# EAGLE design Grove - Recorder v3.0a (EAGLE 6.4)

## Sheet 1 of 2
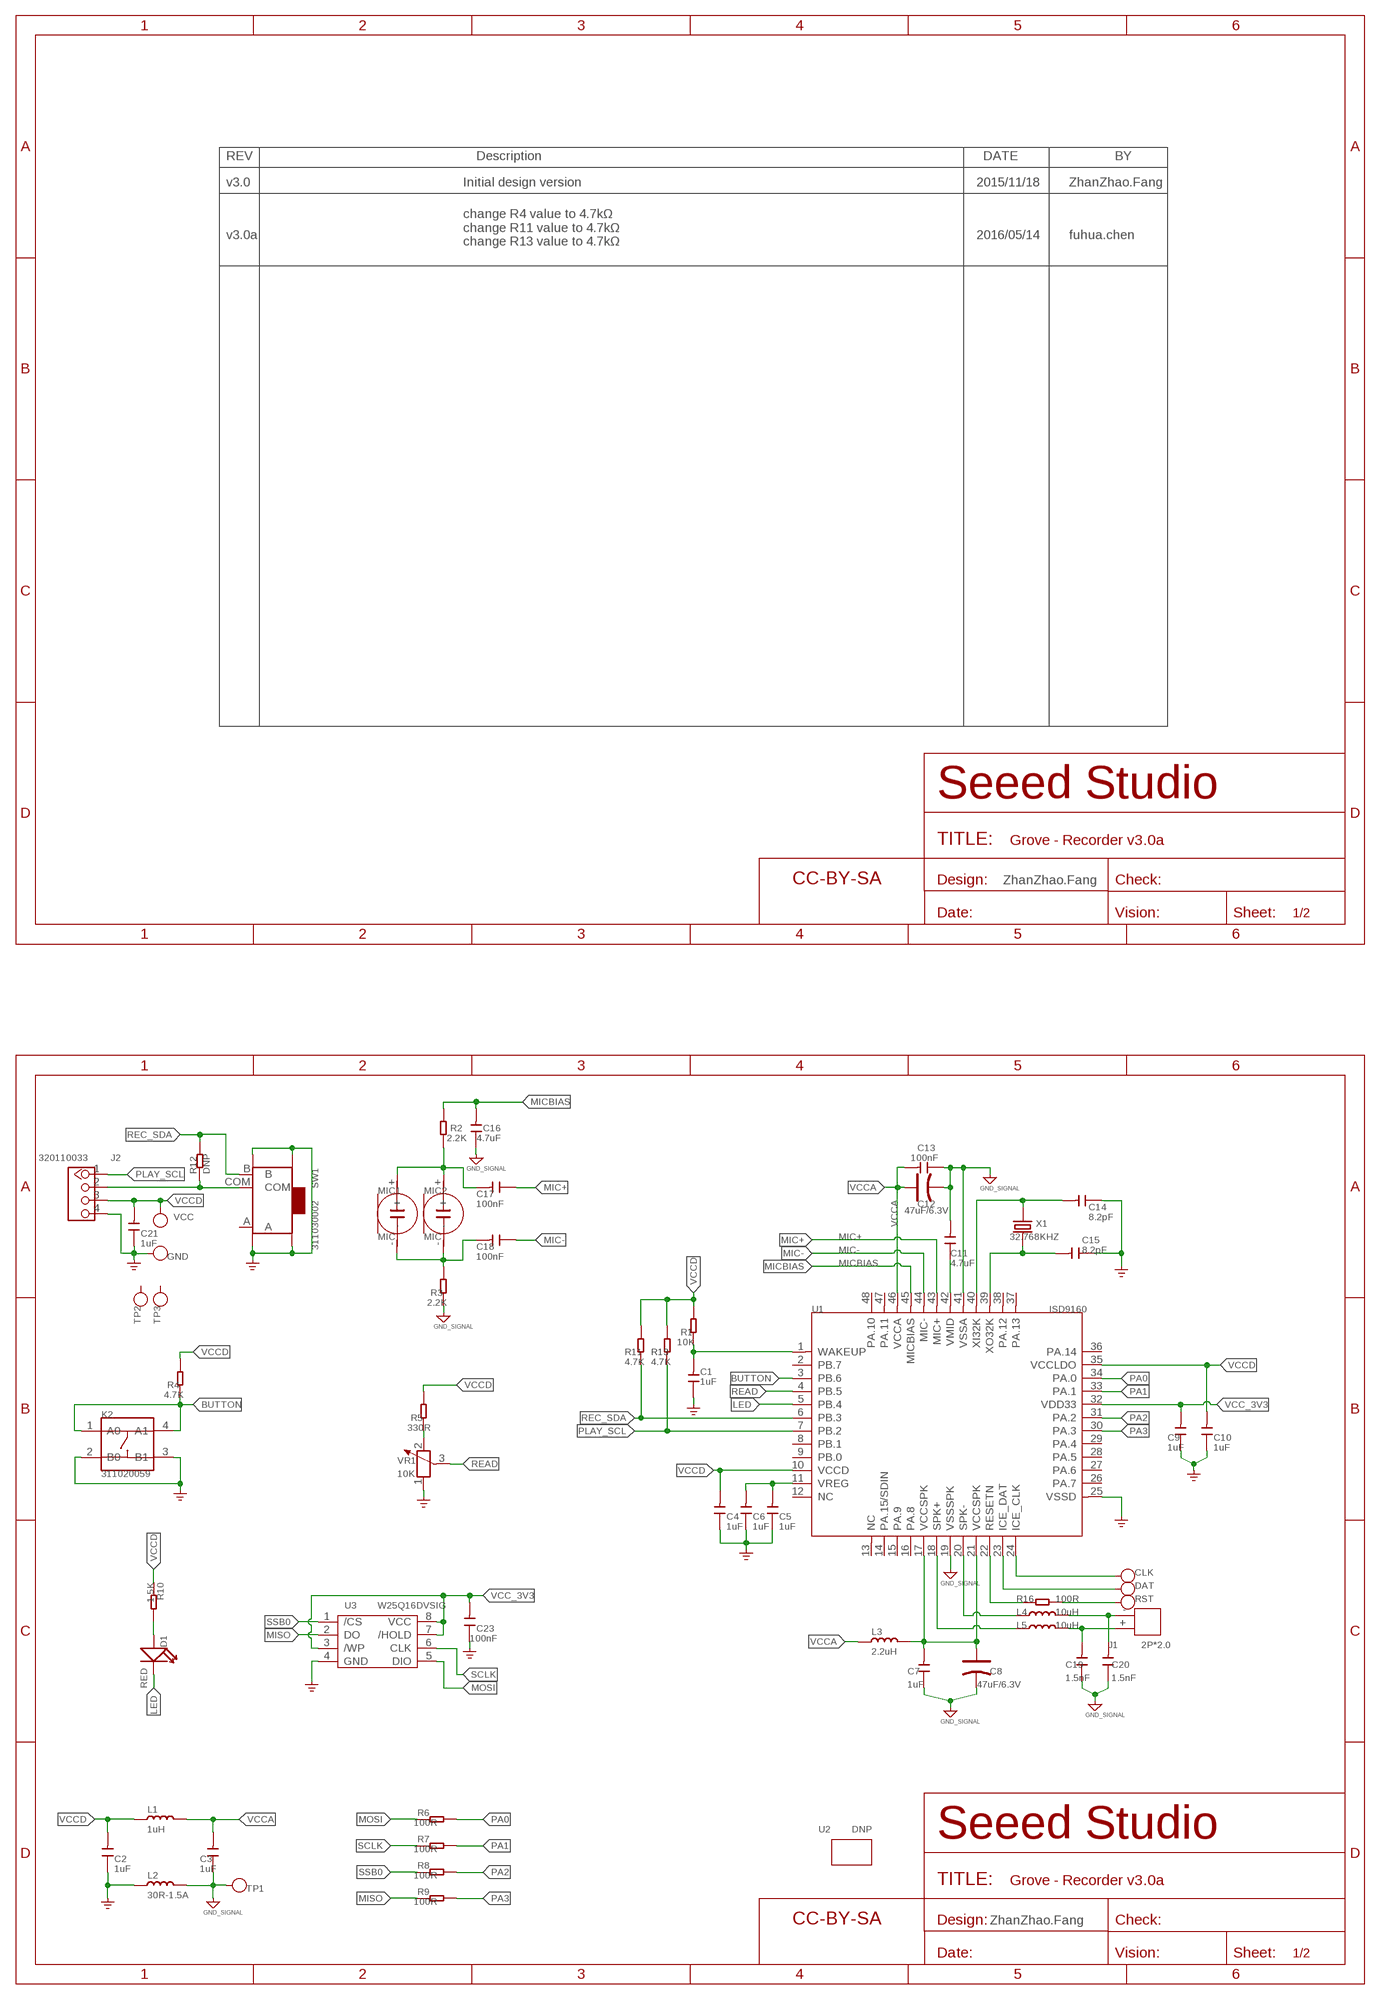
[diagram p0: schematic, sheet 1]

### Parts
C1  1uF  CAP-0603  [C0603]
C2  1uF  CAP-0603  [C0603]
C3  1uF  CAP-0603  [C0603]
C4  1uF  CAP-0603  [C0603]
C5  1uF  CAP-0603  [C0603]
C6  1uF  CAP-0603  [C0603]
C7  1uF  CAP-0603  [C0603]
C8  47uF/6.3V  CAP-POLAR-AVX-A  [AVX-A]
C9  1uF  CAP-0603  [C0603]
C10  1uF  CAP-0603  [C0603]
C11  4.7uF  CAP-0805  [C0805]
C12  47uF/6.3V  CAP-POLAR-AVX-A  [AVX-A]
C13  100nF  CAP-0402  [C0402]
C14  8.2pF  CAP-0402  [C0402]
C15  8.2pF  CAP-0402  [C0402]
C16  4.7uF  CAP-0805  [C0805]
C17  100nF  CAP-0402  [C0402]
C18  100nF  CAP-0402  [C0402]
C19  1.5nF  CAP-0402  [C0402]
C20  1.5nF  CAP-0402  [C0402]
C21  1uF  CAP-0603  [C0603]
C23  100nF  CAP-0402  [C0402]
CLK  DNP  TEST-POINT'4545'  [TP-D45MIL]
D1  RED  LED'RIGHT'  [LED-SIDE-VIEW-0603-RIGHT]
DAT  DNP  TEST-POINT'4545'  [TP-D45MIL]
FR1  DNP  SEEEDSTUDIO-OPEN-SCH-FRAME  [SEEEDSTUDIO-PCB-FRAME]
FR2  DNP  SEEEDSTUDIO-OPEN-SCH-FRAME  [SEEEDSTUDIO-PCB-FRAME]
GND  DNP  TEST-POINT'4545'  [TP-D45MIL]
J1  2P*2.0  JST-2P-DIP'2.0'  [H2-2.0-6X4.5MM]
J2  320110033  GROVE-CONNECTOR-DIP-2.0  [HW4-2.0]
K2  311020059  BUTTON-4P'TS-1109'  [SW4-6.0X6.0X5.0MM]
L1  1uH  INDUCTOR/FERRITE-BEAD'0805'  [L0805]
L2  30R-1.5A  INDUCTOR/FERRITE-BEAD'0603'  [L0603]
L3  2.2uH  INDUCTOR/FERRITE-BEAD'0805'  [L0805]
L4  10uH  INDUCTOR/FERRITE-BEAD'0805'  [L0805]
L5  10uH  INDUCTOR/FERRITE-BEAD'0805'  [L0805]
MIC1  MIC  MIC-2P'EAO-9745-PFA-C1033-28-008'  [MIC2-D9.7XH4.5MM]
MIC2  MIC  MIC-2P'EAO-9745-PFA-C1033-28-008'  [MIC2-D9.7XH4.5MM]
R1  10K  RES-0402  [R0402]
R2  2.2K  RES-0402  [R0402]
R3  2.2K  RES-0402  [R0402]
R4  4.7K  RES-0402  [R0402]
R5  330R  RES-0402  [R0402]
R6  100R  RES-0402  [R0402]
R7  100R  RES-0402  [R0402]
R8  100R  RES-0402  [R0402]
R9  100R  RES-0402  [R0402]
R10  1.5K  RES-0402  [R0402]
R11  4.7K  RES-0402  [R0402]
R12  DNP  RES-0402  [R0402]
R13  4.7K  RES-0402  [R0402]
R16  100R  RES-0402  [R0402]
RST  DNP  TEST-POINT'4545'  [TP-D45MIL]
SW1  311030002  SWITCH-3+4P  [SW7-SMD-L6.7X2.7X3.2MM]
TP1  DNP  TEST-POINT'4545'  [TP-D45MIL]
TP2  DNP  TEST-POINT'4545'  [TP-D45MIL]
TP3  DNP  TEST-POINT'4545'  [TP-D45MIL]
U1  ISD9160  MCU-ISD9160  [LQFP48-0.5-7X7MM]
U2  DNP  GROVE'2U'  [GROVE-1*2-TEST-PLATFORM]
U3  W25Q16DVSIG  FLASH-W25X80  [SOIC8-1.27-5.3X5.3MM]
VCC  DNP  TEST-POINT'4545'  [TP-D45MIL]
VR1  10K  RES-ADJ-SX3362P  [ADJR3-7.0X7.0X5.0MM]
X1  32.768KHZ  CRYSTAL-2P-3215  [X2-SMD-3.2X1.5X0.55MM]

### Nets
AGND: C3.1 C7.1 C8.- C11.2 C12.- C13.1 C16.1 C19.1 C20.1 L2.2 R3.1 TP1.T U1.19(VSSSPK) U1.41(VSSA) ; supply symbol labelled GND_SIGNAL
BUTTON: K2.1(A0) K2.4(A1) R4.1 U1.3(PB.6)
GND: C1.1 C2.1 C4.1 C5.1 C6.1 C9.1 C10.1 C14.1 C15.1 C21.1 C23.1 GND.T J2.4 K2.2(B0) K2.3(B1) L2.1 SW1.SS1 SW1.SS2 SW1.SS3 SW1.SS4 U1.25(VSSD) U3.4(GND) VR1.1 ; supply symbol labelled GND_POWER
ICE_CLK: CLK.T U1.24(ICE_CLK)
LED: D1.2(-) U1.5(PB.4)
MIC+: C17.1 U1.43(MIC+)
MIC-: C18.1 U1.44(MIC-)
MICBIAS: C16.2 R2.2 U1.45(MICBIAS)
MISO: R9.2 U3.2(DO)
MOSI: R6.2 U3.5(DIO)
N$1: C1.2 R1.1 U1.1(WAKEUP)
N$2: C7.2 C8.+ L3.2 U1.17(VCCSPK) U1.21(VCCSPK)
N$3: C5.2 C6.2 U1.11(VREG)
N$4: C11.1 U1.42(VMID)
N$5: C17.2 MIC1.+ MIC2.+ R2.1
N$6: D1.1(+) R10.1
N$7: C14.2 U1.40(XI32K) X1.1
N$8: C15.2 U1.39(XO32K) X1.2
N$9: C18.2 MIC1.- MIC2.- R3.2
N$10: J2.2 R12.2 SW1.COM
N$11: R5.1 VR1.2
N$12: DAT.T U1.23(ICE_DAT)
N$13: L4.1 U1.20(SPK-)
N$16: R16.2 U1.22(RESETN)
N$17: R16.1 RST.T
N$23: L5.1 U1.18(SPK+)
N$24: C20.2 J1.- L4.2
N$25: C19.2 J1.+ L5.2
PA0: R6.1 U1.34(PA.0)
PA1: R7.1 U1.33(PA.1)
PA2: R8.1 U1.31(PA.2)
PA3: R9.1 U1.30(PA.3)
PLAY_SCL: J2.1 R13.1 U1.7(PB.2)
READ: U1.4(PB.5) VR1.3
REC_SDA: R11.1 R12.1 SW1.B U1.6(PB.3)
SCLK: R7.2 U3.6(CLK)
SSB0: R8.2 U3.1(/CS)
VCC_3V3: C9.2 C23.2 U1.32(VDD33) U3.3(/WP) U3.7(/HOLD) U3.8(VCC)
VCCA: C3.2 C12.+ C13.2 L1.2 L3.1 U1.46(VCCA)
VCCD: C2.2 C4.2 C10.2 C21.2 J2.3 L1.1 R1.2 R4.2 R5.2 R10.2 R11.2 R13.2 U1.10(VCCD) U1.35(VCCLDO) VCC.T
Unconnected: SW1.A TP2.T TP3.T U1.2(PB.7) U1.8(PB.1) U1.9(PB.0) U1.12(NC) U1.13(NC) U1.14(PA.15/SDIN) U1.15(PA.9) U1.16(PA.8) U1.26(PA.7) U1.27(PA.6) U1.28(PA.5) U1.29(PA.4) U1.36(PA.14) U1.37(PA.13) U1.38(PA.12) U1.47(PA.11) U1.48(PA.10)

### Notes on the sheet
- v3.0 | Initial design version | 2015/11/18 | ZhanZhao.Fang
- v3.0a | 2016/05/14 | fuhua.chen
- change R4 value to 4.7kΩ
  change R11 value to 4.7kΩ
  change R13 value to 4.7kΩ
- ZhanZhao.Fang
- ZhanZhao.Fang

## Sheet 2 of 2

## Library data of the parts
C1-C7 C9-C11 C13-C21 C23 = Discrete-new:CAP: Ceramic Capacitors
C8 C12 = Discrete-new:CAP-POLAR: Electrolytic Capacitors,Tantalum Capacitors and Super Capacitors
CLK DAT GND RST TP1-TP3 VCC = Discrete-new:TEST-POINT; PARTNO: DNP
D1 = Discrete-new:LED
FR1 FR2 = moudle-new:SEEEDSTUDIO-OPEN-SCH-FRAME
J1 = Connector-new:JST-2P-DIP: 2P-2.0:320110049;2P-2.0-90D:320110027;2P-2.54:320110053;2P-2.54-90D:320110000
J2 = Connector-new:GROVE-CONNECTOR-DIP: 4P-2.0:320110033;4P-2.0-90D:320110034
K2 = Discrete-new:BUTTON-4P: SW4-6.0X6.0X5.0MM:311020024;SW4-8.0X8.0X9.0MM:311020028;SW4-SMD-6.0X6.0X5.0MM:311020004;SW4-SMD-3.35X3.35X1.5MM:311020030;SW4-SMD-5.2X5.2X2.5MM:311020046
L1-L5 = Discrete-new:INDUCTOR/FERRITE-BEAD
MIC1 MIC2 = Discrete-new:MIC-2P: 312030029
R1-R13 R16 = Discrete-new:RES
SW1 = Discrete-new:SWITCH-3+4P: SW7-SMD-6.7X2.6X1.4MM-90D:311030002;SW7-SMD-L6.7X2.7X3.2MM:311030001
U1 = template:MCU-ISD9160
U2 = moudle-new:GROVE
U3 = IC-new:FLASH-W25X80: 1M-BIT,2M-BIT,4M-BIT AND 8M-BIT SERIAL FLASH MEMORY WITH 4KB SECTORS AND DUAL OUTPUT SPI
VR1 = Discrete-new:RES-ADJ: Potentiometer
X1 = Discrete-new:CRYSTAL-2P

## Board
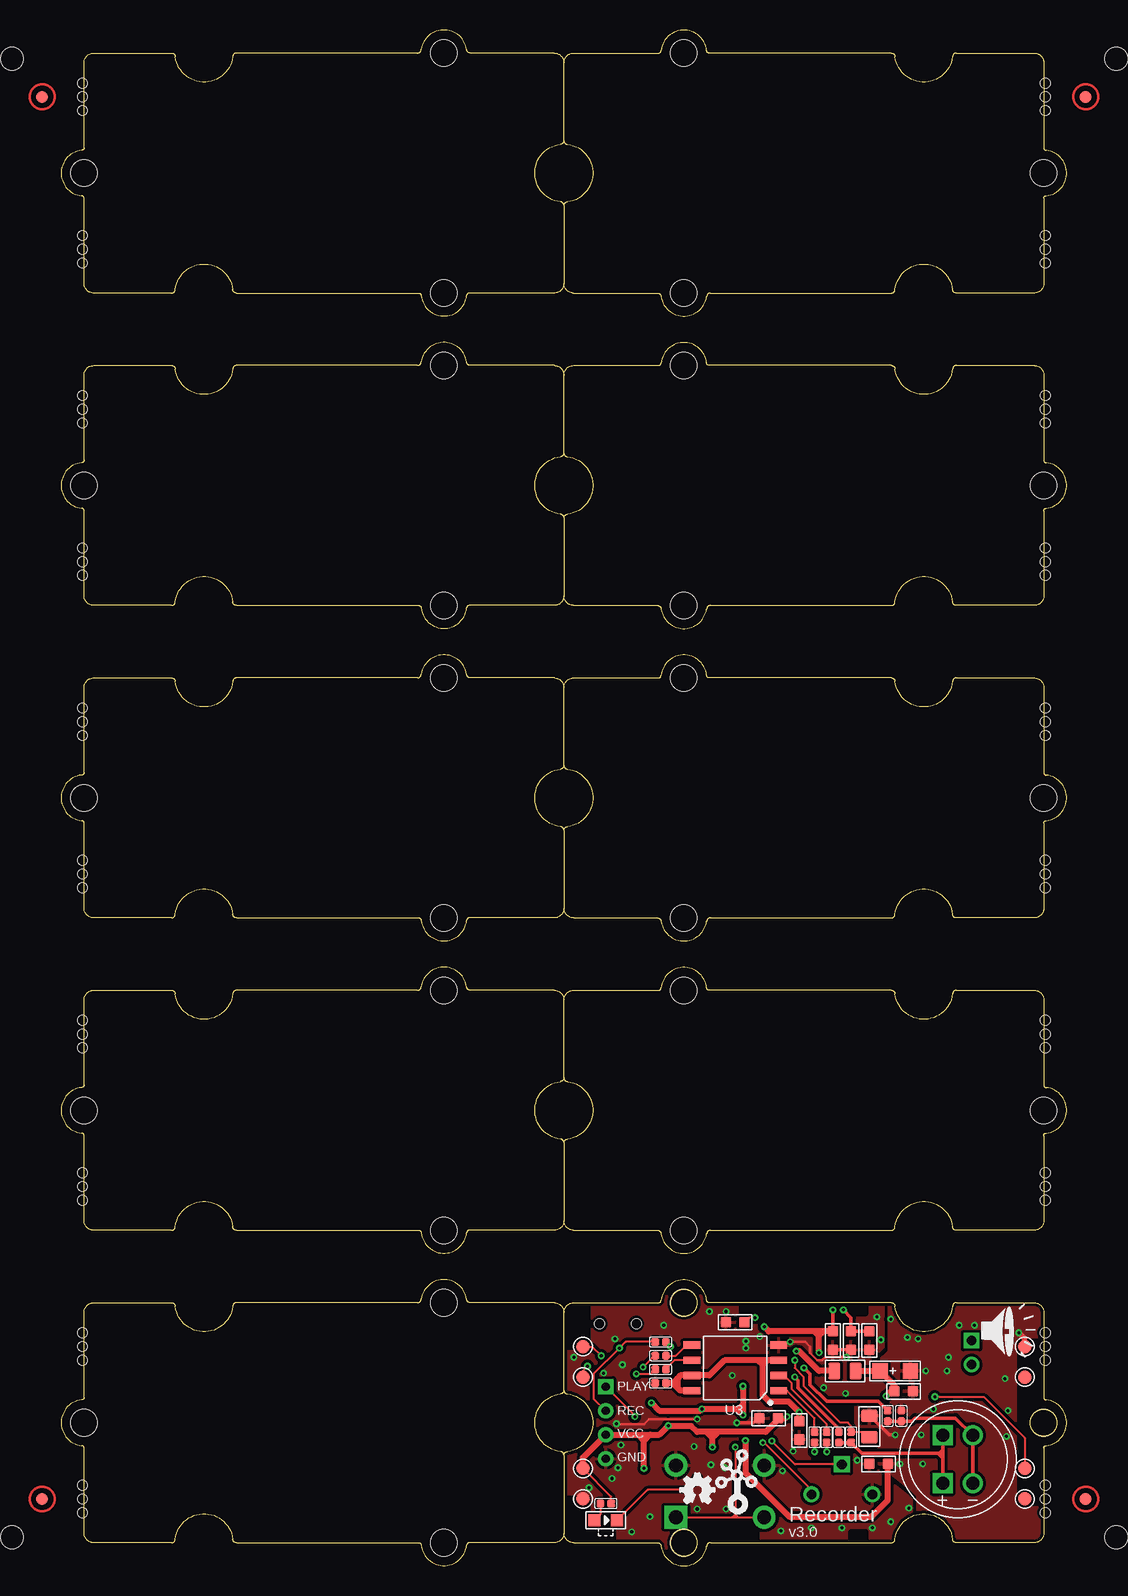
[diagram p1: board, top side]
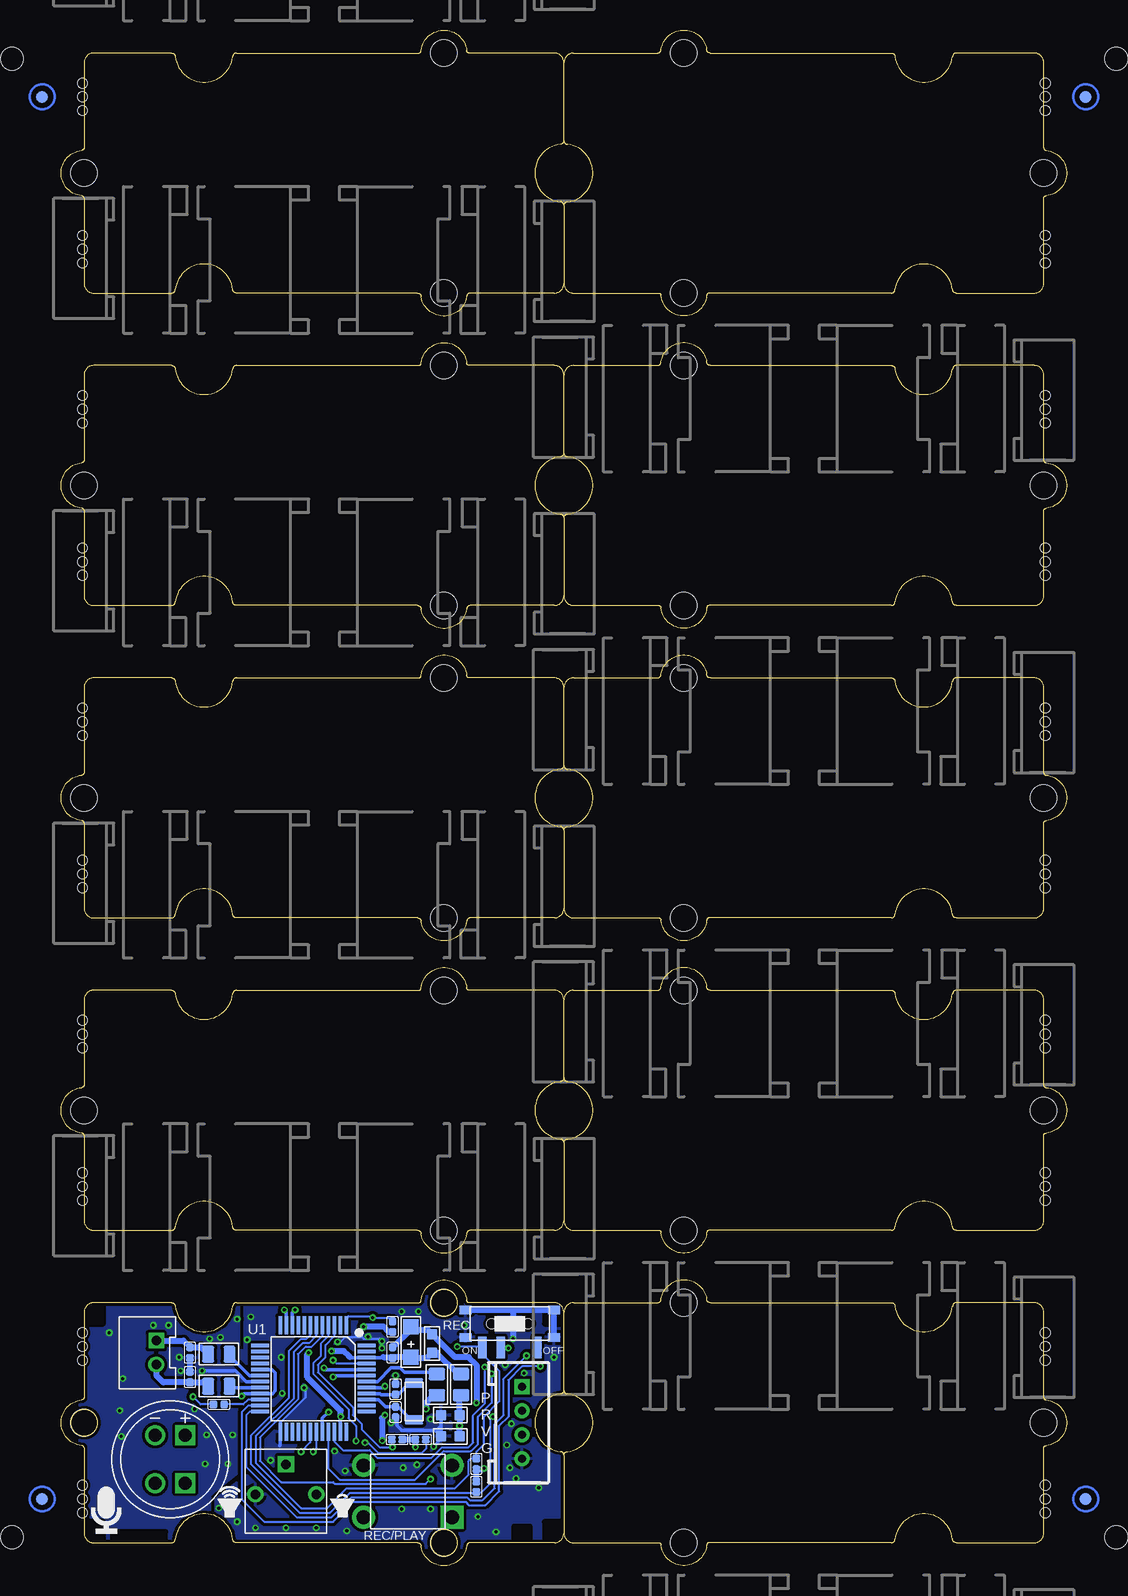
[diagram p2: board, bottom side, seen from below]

Size 83.82 x 127.98 mm. Coordinates in mm from the lower left corner, seen from the top.
Copper layers (1*16): Top 0.035mm / dielectric 1.5mm / Bottom 0.035mm
Design rules "SeeedStudio_2layer_DRU_no_angle_20140221 *": minimum track width 6mil, minimum drill 10mil, track to track 6mil, track to pad 6mil, pad to pad 6mil, via to via 6mil, smd to smd 0mil, copper to edge 10mil, drill to drill 10mil, minimum pad ring 10mil, minimum via ring 6mil, stop-mask expansion 2mil, vias tented up to drill 25mil, thermal gap 10mil
Holes 0.8 mm at 1.78,4.43 1.78,6.71 1.78,5.57 1.78,17.13 1.78,19.41 1.78,18.27 1.78,30.46 1.78,32.75 1.78,31.61 1.78,43.16 1.78,45.45 1.78,44.31 1.78,56.5 1.78,58.78 1.78,57.64 1.78,69.2 1.78,71.48 1.78,70.34 1.78,82.53 1.78,84.82 1.78,83.68 1.78,95.23 1.78,97.52 1.78,96.38 1.78,108.57 1.78,110.85 1.78,109.71 1.78,121.27 1.78,123.55 1.78,122.41 82.04,6.71 82.04,4.43 82.04,5.57 82.04,19.41 82.04,17.13 82.04,18.27 82.04,32.75 82.04,30.46 82.04,31.61 82.04,45.45 82.04,43.16 82.04,44.31 82.04,58.78 82.04,56.5 82.04,57.64 82.04,71.48 82.04,69.2 82.04,70.34 82.04,84.82 82.04,82.53 82.04,83.68 82.04,97.52 82.04,95.23 82.04,96.38 82.04,110.85 82.04,108.57 82.04,109.71 82.04,123.55 82.04,121.27 82.04,122.41
Holes 1.91 mm at -4.13,125.59 87.95,125.59 87.95,2.4 -4.13,2.4
tRestrict: area 44.8,2 to 46,3.3
bRestrict: area 44.8,2 to 46,3.3

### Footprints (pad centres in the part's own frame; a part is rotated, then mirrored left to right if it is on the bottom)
C0603 = smd 0.889 x 0.889: 1 0,0.762; 2 0,-0.762
AVX-A = smd 1.27 x 1.27: + -1.27,0; - 1.27,0
C0805 = smd 1.397 x 1.016: 1 0,0.889; 2 0,-0.889
C0402 = smd 0.635 x 0.635: 1 0,0.445; 2 0,-0.445
TP-D45MIL = smd 1.143 x 1.143: T 0,0
LED-SIDE-VIEW-0603-RIGHT = smd 1 x 1: 1 0,-0.95; 2 0,0.95
H2-2.0-6X4.5MM = drill 0.8 pad 1.3 square: + -1,0.75 | drill 0.8 pad 1.3: - 1,0.75
HW4-2.0 = drill 0.7 pad 1.27 square: 1 -3,0 | drill 0.7 pad 1.27: 2 -1,0; 3 1,0; 4 3,0
SW4-6.0X6.0X5.0MM = drill 1.143 pad 1.905 square: 1 -3.683,2.159 | drill 1.143 pad 1.905: 2 -3.683,-2.159; 3 3.683,-2.159; 4 3.683,2.159
L0805 = smd 1.016 x 1.397: 1 -0.889,0; 2 0.889,0
L0603 = smd 0.889 x 0.889: 1 -0.762,0; 2 0.762,0
MIC2-D9.7XH4.5MM = drill 1.1 square: + 1.25,2 | drill 1.1: - -1.25,2
ROUND-MARK-1.0 = smd 1.016 x 1.016: P$1 0,0
R0402 = smd 0.635 x 0.635: 1 0,0.445; 2 0,-0.445
SW7-SMD-L6.7X2.7X3.2MM = smd 1.8 x 0.7: A 1.978,2.286; B 1.978,-2.286; COM 1.978,-0.762 | smd 0.7 x 1.016: SS1 -1.15,-3.683; SS2 1.15,-3.683; SS3 1.15,3.683; SS4 -1.15,3.683 | hole 0.813: 0,-1.524; 0,1.524
LQFP48-0.5-7X7MM = smd 1.5 x 0.3: 1 -4.45,2.75; 2 -4.45,2.25; 3 -4.45,1.75; 4 -4.45,1.25; 5 -4.45,0.75; 6 -4.45,0.25; 7 -4.45,-0.25; 8 -4.45,-0.75; 9 -4.45,-1.25; 10 -4.45,-1.75; 11 -4.45,-2.25; 12 -4.45,-2.75; 25 4.45,-2.75; 26 4.45,-2.25; 27 4.45,-1.75; 28 4.45,-1.25; 29 4.45,-0.75; 30 4.45,-0.25; 31 4.45,0.25; 32 4.45,0.75; 33 4.45,1.25; 34 4.45,1.75; 35 4.45,2.25; 36 4.45,2.75 | smd 0.3 x 1.5: 13 -2.75,-4.45; 14 -2.25,-4.45; 15 -1.75,-4.45; 16 -1.25,-4.45; 17 -0.75,-4.45; 18 -0.25,-4.45; 19 0.25,-4.45; 20 0.75,-4.45; 21 1.25,-4.45; 22 1.75,-4.45; 23 2.25,-4.45; 24 2.75,-4.45; 37 2.75,4.45; 38 2.25,4.45; 39 1.75,4.45; 40 1.25,4.45; 41 0.75,4.45; 42 0.25,4.45; 43 -0.25,4.45; 44 -0.75,4.45; 45 -1.25,4.45; 46 -1.75,4.45; 47 -2.25,4.45; 48 -2.75,4.45
GROVE-1*2-TEST-PLATFORM = hole 2.2: 10.635,10; 10.635,-10; -19.365,0
SOIC8-1.27-5.3X5.3MM = smd 0.62 x 1.4: 1 -1.905,-3.623; 2 -0.635,-3.623; 3 0.635,-3.623; 4 1.905,-3.623; 5 1.905,3.623; 6 0.635,3.623; 7 -0.635,3.623; 8 -1.905,3.623
GROVE-TEST-PLATFORM = hole 2.2: -10,-10; -10,10; 20,0
ADJR3-7.0X7.0X5.0MM = drill 0.8 pad 1.35: 1 -2.54,-0.25; 2 2.54,-0.25 | drill 0.8 pad 1.35 square: 3 0,2.25
X2-SMD-3.2X1.5X0.55MM = smd 0.762 x 1.524: 1 -1.524,0; 2 1.524,0

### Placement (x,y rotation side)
C1  56.2,20.3 90 top
C2  51.37,12.56 90 bottom
C3  52.9,18.53 0 bottom
C4  64.33,18.78 180 top
C5  67.37,18.78 180 top
C6  65.85,18.78 180 top
C7  70.23,14.52 270 top
C8  69.53,16.24 0 top
C9  61.53,11.29 180 top
C10  58.99,12.3 90 top
C11  52.52,15.1 0 bottom
C12  54.67,18.65 90 bottom
C13  56.2,17.76 0 bottom
C14  55.94,14.72 0 bottom
C15  55.94,12.81 180 bottom
C16  67.37,11.6 0 top
C17  64.83,10.71 0 top
C18  68.9,12.49 0 top
C19  73.09,17.76 180 bottom
C20  73.09,15.73 0 bottom
C21  51.37,10.78 90 bottom
C23  49.98,15.22 90 top
CLK  43.5,18.27 0 top
D1  45.4,3.79 270 top
DAT  43.5,15.73 0 top
FR1  not placed on the board
FR2  not placed on the board
GND  43.5,5.57 0 top
J1  76.65,17.76 270 bottom
J2  45.4,11.92 270 bottom
K2  54.93,6.21 180 bottom
L1  50.48,15.1 90 bottom
L2  68.14,8.49 0 top
L3  65.34,16.24 0 top
L4  70.68,14.97 180 bottom
L5  70.68,17.64 180 bottom
MIC1  74.74,8.87 0 bottom
MIC2  74.74,8.87 180 top
P1  [ROUND-MARK-1.0]  -1.59,122.41 180 bottom
P2  [ROUND-MARK-1.0]  85.41,122.41 180 bottom
P3  [ROUND-MARK-1.0]  -1.59,5.57 180 bottom
P4  [ROUND-MARK-1.0]  85.41,5.57 180 bottom
P5  [ROUND-MARK-1.0]  -1.59,122.41 180 top
P6  [ROUND-MARK-1.0]  85.41,122.41 180 top
P7  [ROUND-MARK-1.0]  85.41,5.57 180 top
P8  [ROUND-MARK-1.0]  -1.59,5.57 180 top
R1  56.2,19.92 0 bottom
R2  65.85,10.71 180 top
R3  70.04,12.49 0 top
R4  55.82,10.52 90 bottom
R5  53.86,10.52 270 bottom
R6  49.98,17.51 90 top
R7  49.98,16.37 90 top
R8  62.8,10.71 180 top
R9  63.82,10.71 180 top
R10  45.4,5.19 90 top
R11  49.21,8.49 0 bottom
R12  49.98,18.65 270 top
R13  49.21,6.59 180 bottom
R16  70.68,13.45 90 bottom
RST  80.33,8.11 0 top
SW1  46.42,20.18 270 bottom
TP1  80.33,18.27 0 top
TP2  80.33,15.73 0 top
TP3  80.33,5.57 0 top
U1  62.8,15.6 270 bottom
U2  62.55,11.92 0 bottom
U3  56.2,16.49 90 top
U4  [GROVE-TEST-PLATFORM]  61.91,90.03 180 bottom
U5  [GROVE-TEST-PLATFORM]  21.91,90.03 0 bottom
U6  [GROVE-TEST-PLATFORM]  61.91,63.99 180 bottom
U7  [GROVE-TEST-PLATFORM]  21.91,63.99 0 bottom
U8  [GROVE-TEST-PLATFORM]  61.91,37.96 180 bottom
U9  [GROVE-TEST-PLATFORM]  21.91,37.96 0 bottom
U10  [GROVE-TEST-PLATFORM]  21.91,11.92 0 bottom
U11  [GROVE-TEST-PLATFORM]  61.91,11.92 180 bottom
U12  [GROVE-TEST-PLATFORM]  61.91,116.06 180 bottom
U13  [GROVE-TEST-PLATFORM]  21.91,116.06 0 bottom
U$20  [TWIGLOGO_SMALL]  54.17,4.17 0 top
U$21  [OSHW_FILLX100_NOTEXT]  51.63,5.19 0 top
VCC  43.5,8.11 0 top
VR1  65.09,6.21 0 bottom
X1  54.42,13.7 270 bottom

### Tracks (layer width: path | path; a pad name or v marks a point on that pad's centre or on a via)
AGND  (via drill 0.25 pad 0.51)
  Top 0.305: C16.1 67.44,12.49 69.03,10.91 v69.53,10.91
  Top 0.406: TP1.T 80.33,18.91 v79.82,19.41
  Top 0.508: v56.83,14.97 56.83,13.45 | 56.83,13.45 v56.83,12.56 56.33,13.06 | 56.33,13.06 v53.4,13.06 53.28,12.94 49.85,12.94 v49.21,13.57 | 56.33,13.06 56.45,13.06 56.83,13.45 | v57.05,10.44 57.05,7.77 60.77,4.05 67.5,4.05 68.9,5.44 L2.2
  Bottom 0.305: U1.41 56.95,14.85 v56.83,14.97 | U1.19 68.39,15.35 69.28,16.24 v72.07,16.24
  Bottom 0.508: C20.1 C19.1 | C13.1 56.13,18.21 54.67,19.67 | C12.- 54.67,19.67 | v56.83,12.56 57.09,12.3 57.09,10.47 v57.05,10.44 | C11.2 52.77,14.21 53.4,13.57 v53.4,13.06 | 54.67,19.67 53.28,19.67 C3.1 50.99,17.38 49.85,17.38 49.21,16.75 v49.21,13.57
  other vias: 78.8,10.78 78.93,12.94 78.68,15.6 76.14,20.05 74.87,20.05 71.44,18.91 70.55,19.03 69.15,20.56 73.85,16.24 73.98,17.38 72.71,13.06 69.91,8.49 71.69,10.91 71.82,8.49
  pour Top (isolate 0.254, rank 2): 82.23,22.46 69.03,22.46 69.03,17.89 68.14,17 66.74,17 66.23,16.49 66.23,10.06 71.06,6.21 71.44,5.83 71.44,1 71.57,0.87 81.6,0.87 82.23,1.51
  pour Bottom (isolate 0.254, rank 2): 82.23,22.46 69.03,22.46 69.03,17.89 68.14,17 66.74,17 66.23,16.49 66.23,10.06 71.06,6.21 71.44,5.83 71.44,1 71.57,0.87 81.6,0.87 82.23,1.51
BUTTON  (via drill 0.25 pad 0.51)
  Top 0.152: v56.2,9.89 56.2,4.3 | 56.2,4.3 56.2,4.05 | K2.1 55.94,4.05 | 55.94,4.05 56.2,4.05 | 56.2,4.05 56.45,4.05 | 56.45,4.05 K2.4 | 56.45,4.05 56.2,4.3 | 56.2,4.3 55.94,4.05
  Bottom 0.152: U1.3 61.05,19.13 61.79,18.4 61.79,17.38 62.42,16.75 62.42,16.11 59.5,13.19 59.5,12.56 58.74,11.79 58.74,11.34 57.29,9.89 v56.2,9.89 56.26,9.95 R4.1
GND  (via drill 0.25 pad 0.51)
  Top 0.203: v53.02,12.23 49.01,12.23 48.58,11.79 46.34,11.79 v46.29,11.85 | v60.77,18.65 62.04,18.65 62.42,18.27 62.42,17.76 63.06,17.13 63.44,17.13 63.69,17.38 v65.47,17.38
  Top 0.305: C10.1 58.1,12.3 57.72,11.92 v56.33,11.92 | v65.47,17.38 65.47,17.51 65.85,17.89 C6.1 C4.1
  Bottom 0.203: v57.09,18.72 57.28,18.91 58.61,18.91 58.74,19.03 60.14,19.03 60.52,18.65 v60.77,18.65 | U1.25 65.55,11.91 63.44,14.03 63.44,14.72 v63.56,14.84
  Bottom 0.305: 55.82,11.92 55.82,11.67 55.44,11.29 52.64,11.29 | 55.82,11.92 55.82,12.24 C15.1 55.94,12.3 v56.33,11.92 55.82,11.92 | U1.25 65.55,10.06 65.6,10.02 | C21.1 52.13,11.29 | 52.13,11.29 52.13,11.67 | 52.13,11.67 C2.1 | 52.64,11.29 C21.1 | 52.52,11.29 52.13,11.29 | 52.64,11.29 52.52,11.29 | 52.52,11.29 52.13,11.67 | C21.1 52.13,10.58 v52.77,9.94
  Bottom 0.508: SW1.SS3 SW1.SS4 | SW1.SS4 | SW1.SS1 46.17,21.33 | 46.17,21.33 SW1.SS4 | 46.17,21.33 46.17,18.91 v46.17,18.91
  other vias: 55.94,15.86 46.42,8.16 44.01,6.51 45.91,7.27 68.01,20.74 68.33,18.83 55.44,21.19 50.23,20.05 42.74,17.38 49.09,4.1 57.09,18.14 54.04,21.19 55.31,8.16 60.14,7.91 66.36,8.8 61.02,9.56 46.67,10.07 46.8,16.75 45.23,16.06 54.17,8.42 65.39,14.36 47.56,2.83 69.15,3.67 67.63,3.16 65.09,3.16 62.55,3.16 55.44,4.73 53.02,4.73 70.68,4.81 60.01,2.9 58.23,19.1
  pour Bottom (isolate 0.254, rank 6): 82.23,22.46 41.59,22.46 41.59,1.51 82.23,1.51
  pour Top (isolate 0.254, rank 6): 82.23,22.46 41.59,22.46 41.59,1.51 82.23,1.51
ICE_CLK  (via drill 0.25 pad 0.51)
  Top 0.152: CLK.T 44.26,18.27 v45.02,17.51
  Bottom 0.152: U1.24 68.09,12.85 68.39,12.56 68.39,8.24 64.2,4.05 61.28,4.05 59.63,5.7 49.98,5.7 49.72,5.44 48.71,5.44 47.69,6.46 47.69,11.79 46.93,12.56 46.93,15.6 v45.02,17.51
LED  (via drill 0.25 pad 0.51)
  Top 0.152: v53.02,7.22 52.13,6.33 48.89,6.33 D1.2
  Bottom 0.152: U1.5 62.05,19.15 62.93,18.27 63.44,18.27 64.07,17.64 64.07,13.88 67.25,10.7 67.25,8.75 65.47,6.97 61.15,6.97 61,6.82 53.43,6.82 v53.02,7.22
MIC+  (via drill 0.25 pad 0.51)
  Top 0.305: C17.1 64.83,11.41 61.41,14.84 61.41,15.48 v61.15,15.73
  Bottom 0.305: U1.43 61.03,15.85 v61.15,15.73
MIC-  (via drill 0.25 pad 0.51)
  Top 0.305: C18.1 68.14,13.7 63.82,13.7 62.42,15.1 62.42,15.99 v61.91,16.49
  Bottom 0.305: U1.44 61.77,16.35 v61.91,16.49
MICBIAS  (via drill 0.25 pad 0.51)
  Top 0.152: v61.15,17.13 61.15,16.49 61.91,15.73 61.91,14.97 64.96,11.92 65.6,11.92 65.85,11.67 R2.2 66.93,11.16 C16.2
  Bottom 0.152: U1.45 60.88,16.85 v61.15,17.13
MISO
  Top 0.152: U3.2 60.26,15.86 60.9,15.22 60.9,14.72 63.82,11.79 R9.2
MOSI
  Top 0.152: U3.5 52.13,18.4 51.25,17.51 R6.2
N$1  (via drill 0.25 pad 0.51)
  Top 0.152: v57.85,20.68 57.34,20.68 C1.2
  Bottom 0.152: U1.1 60.05,20.64 59.88,20.81 57.98,20.81 v57.85,20.68 56.52,20.68 R1.1
N$2  (via drill 0.25 pad 0.51)
  Top 0.508: L3.2 C8.+ 69.47,15.03 C7.2 69.15,14.53 v68.77,14.14
  Bottom 0.305: U1.17 66.23,16.35 65.98,16.1 65.98,14.59 66.21,14.35 U1.21 68.56,14.35 v68.77,14.14
N$3  (via drill 0.25 pad 0.51)
  Top 0.305: C5.2 C6.2 65.85,20.68 v65.22,21.32
  Bottom 0.305: U1.11 65.05,21.16 v65.22,21.32
N$4
  Bottom 0.305: U1.42 57.46,15.35 56.33,16.49 55.56,16.49 55.18,16.11 52.64,16.11 C11.1
N$5
  Top 0.305: C17.2 R2.1 66.74,9.38 73.09,9.38 | 73.22,9.38 73.49,9.38 | MIC2.+ 73.49,9.38 | 73.49,9.38 MIC1.+ | 73.09,9.38 73.22,9.38 | 73.22,9.38 73.47,9.64 | 73.09,9.38 73.47,9
N$6
  Top 0.152: R10.1 44.96,4.3 D1.1
N$7
  Bottom 0.305: U1.40 57.23,14.35 57.15,14.27 C14.2 55.75,14.27 54.8,15.22 X1.1
N$8
  Bottom 0.305: X1.2 54.67,12.18 55.75,13.26 C15.2 56.77,13.26 57.37,13.85 U1.39
N$9
  Top 0.305: MIC2.- MIC1.- 74.56,12.3 71.18,12.3 70.93,12.05 R3.2 C18.2
N$10  (via drill 0.25 pad 0.51)
  Top 0.152: 45.4,12.94 J2.2 44.39,13.94 44.39,15.99 v46.55,18.14 47.05,18.65 R12.2
  Bottom 0.152: SW1.COM 46.6,18.2 v46.55,18.14
N$11  (via drill 0.25 pad 0.51)
  Top 0.152: VR1.2 62.55,6.33 58.61,10.27 v58.48,10.27
  Bottom 0.152: R5.1 53.42,9.75 53.79,9.38 57.34,9.38 58.23,10.27 v58.48,10.27
N$12  (via drill 0.25 pad 0.51)
  Top 0.152: DAT.T 43.5,16.24 v43.88,16.62
  Bottom 0.152: U1.23 68.23,13.35 68.77,12.81 68.77,5.55 66.88,3.67 61.15,3.67 59.5,5.32 50.1,5.32 49.85,5.06 48.45,5.06 47.31,6.21 47.31,11.67 46.55,12.43 46.55,15.48 45.4,16.62 v43.88,16.62
N$13
  Bottom 0.305: U1.20 69.67,14.85 L4.1
N$16
  Bottom 0.152: U1.22 68.24,13.85 68.64,13.45 R16.2
N$17  (via drill 0.25 pad 0.51)
  Top 0.152: v72.84,14.08 76.9,14.08 80.33,10.65 RST.T
  Bottom 0.152: R16.1 72.2,13.45 v72.84,14.08
N$23
  Bottom 0.305: U1.18 68.13,15.85 69.79,17.51 L5.1
N$24
  Bottom 0.508: J1.- 75.9,15.87 75.31,15.29 C20.2 71.88,15.29 L4.2
N$25
  Bottom 0.508: L5.2 72.14,18.21 C19.2 73.65,18.76 J1.+
PA0  (via drill 0.25 pad 0.51)
  Top 0.152: v48.51,16.56 49.47,17.51 R6.1
  Bottom 0.152: U1.34 61.05,10.36 60.32,9.64 58.1,9.64 57.47,9 52.95,9 52.08,9.86 49.87,9.86 49.47,10.27 49.47,12.56 48.51,13.51 v48.51,16.56
PA1  (via drill 0.25 pad 0.51)
  Top 0.152: v47.94,15.99 49.15,15.99 R7.1
  Bottom 0.152: U1.33 61.55,8.13 60.59,7.17 54.32,7.17 51.93,9.56 49.67,9.56 49.09,10.14 49.09,12.43 47.94,13.57 v47.94,15.99
PA2  (via drill 0.25 pad 0.51)
  Top 0.152: R8.1 v62.8,9.51
  Bottom 0.152: v62.8,9.51 62.55,9.76 62.55,9.77 U1.31
PA3  (via drill 0.25 pad 0.51)
  Top 0.152: R9.1 v63.82,9.51
  Bottom 0.152: v63.82,9.51 63.05,10.27 U1.30
PLAY_SCL  (via drill 0.25 pad 0.51)
  Top 0.152: J2.1 47.82,12.51 v47.82,12.43
  Bottom 0.152: U1.7 63.05,19.22 63.06,19.22 63.37,18.91 63.82,18.91 64.86,17.87 64.86,13.98 68.01,10.83 68.01,8.49 63.95,4.43 61.41,4.43 59.75,6.08 49.28,6.08 R13.1 48.77,6.14 48.07,6.84 48.07,12.18 v47.82,12.43
READ  (via drill 0.25 pad 0.51)
  Top 0.152: VR1.3 61.19,8.46 v59.25,10.4
  Bottom 0.152: U1.4 61.55,19.14 62.17,18.53 62.17,17.51 62.8,16.87 62.8,15.99 59.88,13.06 59.88,12.3 59.25,11.67 v59.25,10.4
REC_SDA  (via drill 0.25 pad 0.51)
  Top 0.152: R12.1 v50.8,18.27
  Bottom 0.152: U1.6 62.55,19.16 63.13,18.58 63.64,18.58 64.44,17.78 64.44,13.94 67.6,10.78 67.6,8.59 63.82,4.81 61.66,4.81 60.01,6.46 50.99,6.46 49.85,7.6 49.85,8.75 49.66,8.94 R11.1 49.21,9.51 48.58,10.14 48.58,12.43 47.31,13.7 47.31,16.24 48.71,17.64 48.71,18.14 | SW1.B 48.71,18.14 | 48.71,18.14 48.83,18.27 v50.8,18.27
SCLK
  Top 0.152: R7.2 50.42,16.43 51.12,17.13 U3.6
SSB0
  Top 0.152: R8.2 62.8,12.3 60.52,14.59 U3.1
VCC_3V3  (via drill 0.25 pad 0.51)
  Top 0.508: 58.48,16.75 58.48,14.21 58.99,13.7 60.64,13.7 v61.53,12.81 C9.2 | 58.48,16.75 58.48,17.13 | U3.8 51.63,14.59 51.37,14.84 | 51.37,15.6 51.63,15.86 U3.7 54.04,15.86 55.31,17.13 58.1,17.13 | 51.37,15.6 51.37,15.22 | 51.37,15.22 51.37,14.84 | U3.3 58.87,17.13 | 58.87,17.13 58.48,17.13 | 58.48,17.13 58.1,17.13 | 58.48,16.75 58.87,17.13 | 58.48,16.75 58.1,17.13 | 51.37,15.22 50.99,15.22 | 50.99,15.22 C23.2 | 50.99,15.22 51.37,15.6 | 50.99,15.22 51.37,14.84
  Bottom 0.305: U1.32 62.05,12.29 v61.53,12.81
VCCA  (via drill 0.25 pad 0.51)
  Top 0.508: L3.1 63.18,16.24 61.53,17.89 v61.28,17.89
  Bottom 0.305: 56.96,17.38 56.99,17.35 U1.46 59.73,17.35 59.88,17.51
  Bottom 0.508: C12.+ 56.13,17.38 C13.2 56.26,17.38 56.96,17.38 | 59.75,17.38 59.88,17.51 60.26,17.89 v61.28,17.89 | L1.2 50.74,15.99 52.52,17.76 C3.2 53.34,17.32 54.61,17.32
  Bottom 0.61: 54.61,17.32 C12.+
VCCD  (via drill 0.25 pad 0.51)
  Top 0.152: R10.2 45.85,5.76 VCC.T
  Top 0.305: C4.2 v64.33,21.32
  Top 0.508: v60.52,12.43 60.39,12.3 C10.2 59.75,12.18 58.74,11.16 54.8,11.16 | 48.45,10.92 J2.3 43.5,9.02 VCC.T | 48.45,10.92 49.1,10.92 | 49.1,10.92 49.86,10.92 v50.61,11.67 52.52,11.67 53.02,11.16 53.79,11.16 | 54.8,11.16 54.29,11.16 | 54.29,11.16 53.79,11.16 | v54.29,9.89 54.29,10.65 | 54.29,10.65 54.29,11.16 | 54.29,10.65 54.8,11.16 | 54.29,10.65 53.79,11.16 | v48.58,8.11 48.58,10.4 | 48.58,10.4 48.58,10.79 48.45,10.92 | 49.1,10.92 48.58,10.4 | 48.58,10.4 48.07,10.91 | C4.2 63.56,19.54 | 63.56,19.54 63.18,19.54 | 63.18,19.54 62.8,19.54 | 62.8,19.54 58.99,19.54 v58.61,19.92 | v63.18,17.76 63.18,19.16 | 63.18,19.16 63.18,19.54 | 63.18,19.16 63.56,19.54 | 63.18,19.16 62.8,19.54
  Bottom 0.305: U1.10 64.55,21.09 v64.33,21.32 | U1.35 60.55,12.39 v60.52,12.43
  Bottom 0.508: v60.52,12.43 60.52,12.94 63.31,15.73 63.31,17.64 v63.18,17.76 | C21.2 v50.61,11.67 C2.2 50.61,14.08 L1.1 | v54.29,9.89 54.31,9.9 R5.2 R4.2 | v48.58,8.11 48.64,8.05 R11.2 R13.2 | R1.2 56.52,19.48 56.96,19.92 v58.61,19.92

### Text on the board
tPlace: PLAY | REC | VCC | GND | Recorder | v3.0
bPlace: REC | OFF | ON | P | R | V | G | REC/PLAY

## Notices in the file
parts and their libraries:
moudle-new: This work is licensed under the Creative Commons Attribution 4.0 International License.
To view a copy of this license,visit:
http://creativecommons.org/licenses/by-sa/4.0
moudle-new: CC-BY-SA
